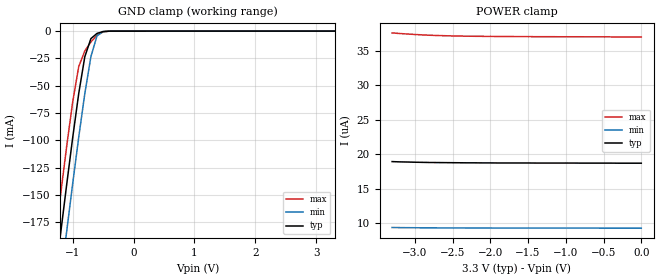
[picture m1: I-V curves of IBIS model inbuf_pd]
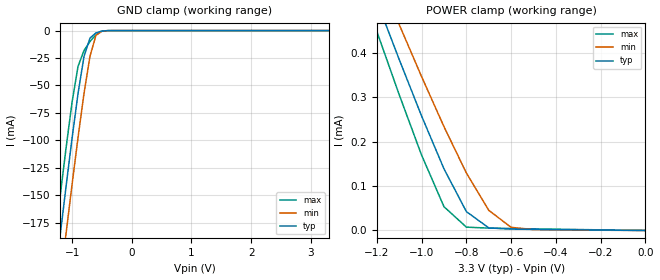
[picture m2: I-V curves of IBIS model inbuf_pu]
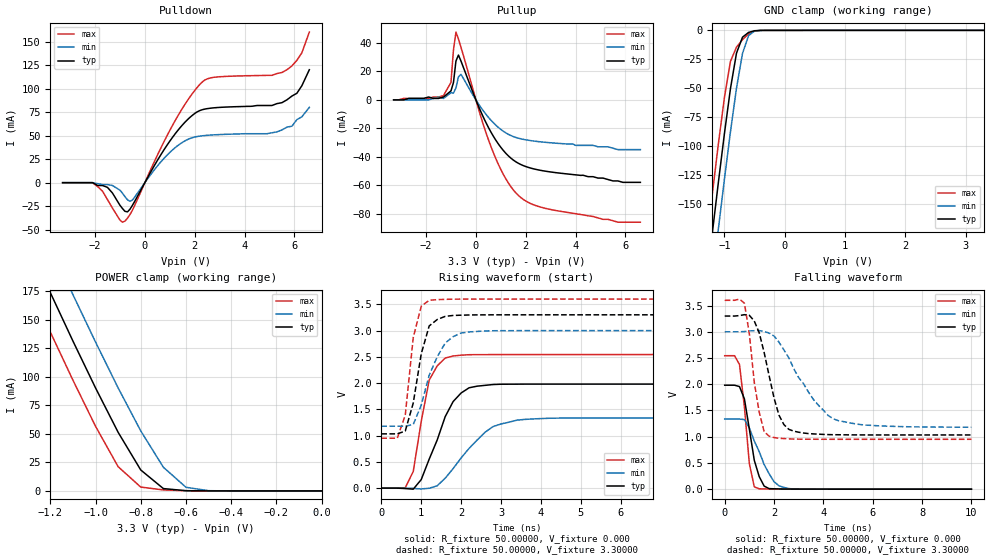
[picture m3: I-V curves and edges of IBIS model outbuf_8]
| IBIS file idt23s08e_8.ibs created by s2ibis2 version 1.2
| North Carolina State University Electronics Research Laboratory  1995
[IBIS ver]   2.1
[File name]   idt23s08e_8.ibs
[File Rev]   2.1
[Date]   Thursday, August 25 , 2005
[Source]   IDT
[Notes]   1. Temp typ=25C, min=-40C, max=100C
   2. IDT 0.5 process
   3. Ramp rates based on 50 ohm load
[Disclaimer]
Integrated Device Technology, Inc. ("IDT") hereby grants the user of this
IBIS model ("User") a non-exclusive, nontransferable license to use this
IBIS model under the following terms: The User is granted this license only
to use the IBIS model for demonstration purposes only and is not granted
rights to sell, copy (except as needed to run the IBIS model), rent, lease
or sub-license (except for demonstration) the IBIS model in whole or in
part, or in modified form to anyone. The User may modify the IBIS model to
suit its specific applications, but  rights to derivative works and such
modifications shall belong to IDT.
THIS IBIS MODEL IS PROVIDED ON AN AS IS" BASIS AND IDT  MAKES ABSOLUTELY NO
WARRANTY WITH RESPECT TO THE INFORMATION CONTAINED HEREIN.  IDT DISCLAIMS
AND USER WAIVES ALL WARRANTIES, EXPRESS AND IMPLIED, INCLUDING WARRANTIES OF
MERCHANTABILITY AND FITNESS FOR A PARTICULAR PURPOSE.  THE ENTIRE RISK AS TO
QUALITY AND PERFORMANCE IS WITH THE USER  ACCORDINGLY, IN NO EVENT SHALL IDT
BE LIABLE FOR ANY DIRECT OR INDIRECT DAMAGES, WHETHER IN CONTRACT OR TORT,
INCLUDING ANY LOST PROFITS OR OTHER INCIDENTAL, CONSEQUENTIAL, EXEMPLARY, OR
PUNITIVE DAMAGES ARISING OUT OF THE USE OR APPLICATION OF THE  IBIS MODEL,
WHETHER OR NOT IDT HAD NOTICE OF SUCH DAMAGES.
IDT reserves the right to make changes without notice to any product herein
to improve reliability, function, or design. IDT does not convey any license
under patent rights or any other intellectual property rights, including
those of third parties. IDT is not obligated to provide maintenance or
support for the licensed IBIS model.
*This model is for the 3.3V Zero Delay Clock Multiplier, Spread Spectrum
*Compatible
[Copyright]
Copyright 2002, Integrated Device Technology, Inc. All rights reserved.
|History
|Rev 1.0 Created on October 21 2003
|   2.0 Regenerated file on August 18 2005
|   2.1 GND and POWER clamp current with a 2ohm resistor in series with
|   pin to simulate diode resistance August 25 2005
|   Component IDT23S08E
[Component]   IDT23S08E
[Manufacturer]   Integrated Device Technology, Inc.
[Package]
|SO16-10 (Thin Shrink Size Outline Package)
| variable   typ   min   max
R_pkg   52.59m   52.19m   52.96m
L_pkg   4.36nH   3.91nH   4.78nH
C_pkg   0.24pF   0.22pF   0.29pF
|SO16-8 (Small Outline Package)
|[R_pkg]   53.14m   52.77m   53.55m
|[L_pkg]   5.18nH   4.04nH   6.38nH
|[C_pkg]   0.38pF   0.224pF   0.551pF
[Pin]  signal_name   model_name   R_pin   L_pin   C_pin
1   REF   inbuf_pd
2   CLKA1   outbuf_8
3   CLKA2   outbuf_8
4   VDD   POWER
5   GND   GND
6   CLKB1   outbuf_8
7   CLKB2   outbuf_8
8   S2   inbuf_pu
9   S1   inbuf_pu
10   CLKA1   outbuf_8
11   CLKA2   outbuf_8
12   GND   GND
13   VDD   POWER
14   CLKA1   outbuf_8
15   CLKA2   outbuf_8
16   CLKOUT   outbuf_8
| Models and submodels in the file (3): inbuf_pd (Input), inbuf_pu (Input), outbuf_8 (3-state)
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| d   d   dummy_model
| oe   oe   dummy_model
|   Model inbuf_pd
[Model]   inbuf_pd
Model_type   Input
Vinl =  0.80000V
Vinh =  2.00000V
C_comp   5.25000pF   5.25000pF   5.25000pF
[Temperature Range]   25.00000   100.00000   -40.00000
[Voltage Range]   3.30000V   3.00000V   3.60000V
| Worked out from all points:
|   GND clamp passes 1 mA (typ) near -0.54 V on its own axis
[GND_clamp]
| voltage   I(typ)   I(min)   I(max)
-3.3V     -1.185A    -1.225A    -1.151A
-1.3V     -232.4mA   -275.4mA   -196.4mA
-1.2V     -186.6mA   -229.6mA   -150.8mA
-1.1V     -141.6mA   -184.4mA   -106.5mA
-1V       -98mA      -140.1mA   -65.13mA
-900mV    -57.16mA   -97.22mA   -32.53mA
-800mV    -23.43mA   -57.16mA   -18.11mA
-700mV    -6.867mA   -23.35mA   -9.97mA
-600mV    -2.108mA   -4.373mA   -3.788mA
-500mV    -376.3uA   -455.1uA   -637.4uA
-400mV    -39.97uA   -43.59uA   -54.23uA
3.3V      18.7uA     9.282uA    36.99uA
[POWER_clamp]
| voltage   I(typ)   I(min)   I(max)
-3.3V     18.93uA    9.375uA    37.59uA
-3.2V     18.89uA    9.361uA    37.5uA
-3V       18.84uA    9.34uA     37.36uA
-2.8V     18.8uA     9.325uA    37.25uA
-2.5V     18.77uA    9.311uA    37.15uA
-2.3V     18.75uA    9.305uA    37.11uA
-1.8V     18.73uA    9.297uA    37.06uA
-1.5V     18.73uA    9.293uA    37.05uA
-1.4V     18.72uA    9.292uA    37.04uA
-900mV    18.72uA    9.288uA    37.03uA
-800mV    18.71uA    9.287uA    37.03uA
0V        18.7uA     9.279uA    37uA
|   Model inbuf_pu
[Model]   inbuf_pu
Model_type   Input
Vinl =  0.80000V
Vinh =  2.00000V
C_comp   5.25000pF   5.25000pF   5.25000pF
[Temperature Range]   25.00000   100.00000   -40.00000
[Voltage Range]   3.30000V   3.00000V   3.60000V
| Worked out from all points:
|   GND clamp passes 1 mA (typ) near -0.54 V on its own axis
|   POWER clamp passes 1 mA (typ) near -1.56 V on its own axis
[GND_clamp]
| voltage   I(typ)   I(min)   I(max)
-3.3V     -1.185A    -1.225A    -1.151A
-1.3V     -232.4mA   -275.4mA   -196.4mA
-1.2V     -186.6mA   -229.6mA   -150.8mA
-1.1V     -141.6mA   -184.4mA   -106.5mA
-1V       -98mA      -140.1mA   -65.13mA
-900mV    -57.16mA   -97.22mA   -32.53mA
-800mV    -23.43mA   -57.16mA   -18.11mA
-700mV    -6.865mA   -23.35mA   -9.967mA
-600mV    -2.105mA   -4.372mA   -3.785mA
-500mV    -373.2uA   -453.1uA   -633.1uA
-400mV    -37.63uA   -42.04uA   -50.7uA
3.3V      26pA       932.9nA    -1.919uA
[POWER_clamp]
| voltage   I(typ)   I(min)   I(max)
-3.3V     3.436mA    3.233mA    3.639mA
-1.3V     650.7uA    705.6uA    594.8uA
-1.2V     516.8uA    584uA      448.6uA
-1.1V     385.3uA    464.1uA    305.8uA
-1V       257.9uA    346.7uA    169.7uA
-900mV    138.8uA    233.9uA    53.5uA
-800mV    42.53uA    129.4uA    7.547uA
-700mV    5.822uA    45.39uA    5.256uA
-600mV    3.108uA    7.059uA    4.42uA
-500mV    2.493uA    1.92uA     3.634uA
0V        25.99pA    392.8pA    1.378pA
|   Model outbuf_8
[Model]   outbuf_8
Model_type   3-state
Polarity   Non-Inverting
Enable   Active-High
Vmeas =  1.650000V
C_comp   7.00000pF   7.00000pF   7.00000pF
[Temperature Range]   25.00000   100.00000   -40.00000
[Voltage Range]   3.30000V   3.00000V   3.60000V
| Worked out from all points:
|   slope of the pulldown table from 0 to 0.495 V, typ, clamps not added: 21.3 ohm
|   slope of the pullup table from 0 to 0.495 V, typ, clamps not added: 25.9 ohm
|   GND clamp passes 1 mA (typ) near -0.55 V on its own axis
|   POWER clamp passes 1 mA (typ) near -0.64 V on its own axis
|   rising waveform, R_fixture 50.00000, V_fixture 0.000: 20-80 % time 636ps typ, 922ps min, 354ps max; typ from 0 V to 1.98 V
|   rising waveform, R_fixture 50.00000, V_fixture 3.30000: 20-80 % time 359ps typ, 524ps min, 256ps max; typ from 1.03 V to 3.3 V
|   falling waveform, R_fixture 50.00000, V_fixture 0.000: 20-80 % time 452ps typ, 757ps min, 311ps max; typ from 1.98 V to 0 V
|   falling waveform, R_fixture 50.00000, V_fixture 3.30000: 20-80 % time 683ps typ, 1.49ns min, 433ps max; typ from 3.3 V to 1.03 V
[Pulldown]
| voltage   I(typ)   I(min)   I(max)
-3.3V     0A         0A         0A
-2.1V     0A         0A         0A
-1.5V     -5mA       -2mA       -18mA
-1V       -24mA      -8mA       -39.7mA
-800mV    -30.4mA    -14.8mA    -40.87mA
-500mV    -24.16mA   -18.47mA   -29.3mA
1.2V      51.36mA    36.85mA    65.17mA
2.2V      76.56mA    49.44mA    104.3mA
2.8V      79.59mA    50.85mA    112.1mA
5.5V      85mA       56mA       117mA
6.1V      95mA       67mA       130mA
6.6V      120mA      80mA       160mA
[Pullup]
| voltage   I(typ)   I(min)   I(max)
-3.3V     0A         0A         0A
-1.3V     2mA        1mA        3mA
-1V       6.3mA      5mA        12.3mA
-900mV    12.2mA     4.8mA      35.1mA
-800mV    27.32mA    8.4mA      47.64mA
-700mV    31.49mA    16.13mA    42.76mA
-600mV    27.33mA    17.93mA    37.06mA
600mV     -22.54mA   -14.21mA   -32.63mA
1.1V      -35.56mA   -22.07mA   -52.35mA
1.6V      -43.51mA   -26.41mA   -65.33mA
2.8V      -50.17mA   -29.87mA   -76.32mA
6.6V      -58mA      -35mA      -86mA
[GND_clamp]
| voltage   I(typ)   I(min)   I(max)
-3.3V     -1.149A    -1.186A    -1.117A
-1.3V     -219.8mA   -260.1mA   -185.9mA
-1.2V     -175.2mA   -215.6mA   -141.4mA
-1.1V     -131.6mA   -171.8mA   -98.29mA
-1V       -89.45mA   -129mA     -58.05mA
-900mV    -50.47mA   -87.86mA   -26.91mA
-800mV    -19.75mA   -50.09mA   -14.52mA
-700mV    -5.912mA   -19.93mA   -8.033mA
-600mV    -1.786mA   -4.555mA   -3.096mA
-500mV    -324uA     -573.1uA   -535.2uA
-400mV    -35.4uA    -49.21uA   -47.52uA
3.3V      18.42uA    10.23uA    36.55uA
[POWER_clamp]
| voltage   I(typ)   I(min)   I(max)
-3.3V     1.109A     1.147A     1.078A
-1.3V     216.7mA    257.2mA    182.3mA
-1.2V     173.7mA    214.3mA    139.2mA
-1.1V     131.3mA    171.9mA    97.06mA
-1V       90.24mA    130.4mA    56.63mA
-900mV    51.34mA    90.22mA    21.24mA
-800mV    18.35mA    52.57mA    3.384mA
-700mV    2.067mA    20.75mA    862.6uA
-600mV    211.3uA    3.195mA    172.4uA
-500mV    44.27uA    214.9uA    51.86uA
0V        18.42uA    9.13uA     36.56uA
[Ramp]
| variable   typ   min   max
dV/dt_r   1.18860/0.56242n   0.80160/0.91807n   1.52580/0.35218n
dV/dt_f   1.35960/0.66169n   1.09140/1.49060n   1.58910/0.36716n
R_load = 50.00000
[Rising Waveform]
R_fixture = 50.00000
V_fixture = 0.000
V_fixture_min = 0.000
V_fixture_max = 0.000
| time   V(typ)   V(min)   V(max)
0s        0V         0V         0V
600ps     -8.128mV   -228.1uV   7.613mV
800ps     -19.72mV   -5.364mV   317mV
1.2ns     552.6mV    -2.433mV   2.056V
1.6ns     1.36V      188.1mV    2.476V
1.8ns     1.649V     372.8mV    2.515V
2.2ns     1.911V     757.2mV    2.539V
2.8ns     1.972V     1.171V     2.542V
3.4ns     1.979V     1.294V     2.542V
10ns      1.981V     1.336V     2.543V
[Rising Waveform]
R_fixture = 50.00000
V_fixture = 3.30000
V_fixture_min = 3.00000
V_fixture_max = 3.60000
| time   V(typ)   V(min)   V(max)
0s        1.033V     1.179V     950.5mV
400ps     1.033V     1.179V     950.5mV
600ps     1.087V     1.179V     1.389V
800ps     1.62V      1.211V     2.867V
1ns       2.556V     1.579V     3.462V
1.2ns     3.088V     2.15V      3.576V
1.6ns     3.269V     2.761V     3.594V
1.8ns     3.287V     2.884V     3.597V
2.2ns     3.296V     2.973V     3.599V
10ns      3.299V     2.999V     3.599V
[Falling Waveform]
R_fixture = 50.00000
V_fixture = 0.000
V_fixture_min = 0.000
V_fixture_max = 0.000
| time   V(typ)   V(min)   V(max)
0s        1.981V     1.336V     2.543V
400ps     1.981V     1.336V     2.543V
600ps     1.955V     1.336V     2.376V
800ps     1.719V     1.326V     1.562V
1ns       1.142V     1.166V     483.6mV
1.2ns     548.3mV    917.7mV    43.61mV
1.6ns     57.95mV    469.1mV    5.853mV
2ns       7.197mV    141.9mV    2.239mV
2.6ns     2.167mV    10.64mV    837.9uV
10ns      42.33uV    45.76uV    52.61uV
[Falling Waveform]
R_fixture = 50.00000
V_fixture = 3.30000
V_fixture_min = 3.00000
V_fixture_max = 3.60000
| time   V(typ)   V(min)   V(max)
0s        3.299V     2.999V     3.599V
800ps     3.325V     3.004V     3.543V
1.4ns     2.979V     3.022V     1.466V
1.6ns     2.603V     3.006V     1.095V
1.8ns     2.164V     2.974V     1.01V
2.2ns     1.41V      2.8V       970.3mV
2.6ns     1.14V      2.503V     958.9mV
3.6ns     1.053V     1.708V     951.2mV
4.4ns     1.038V     1.341V     950.6mV
10ns      1.033V     1.18V      950.5mV
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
